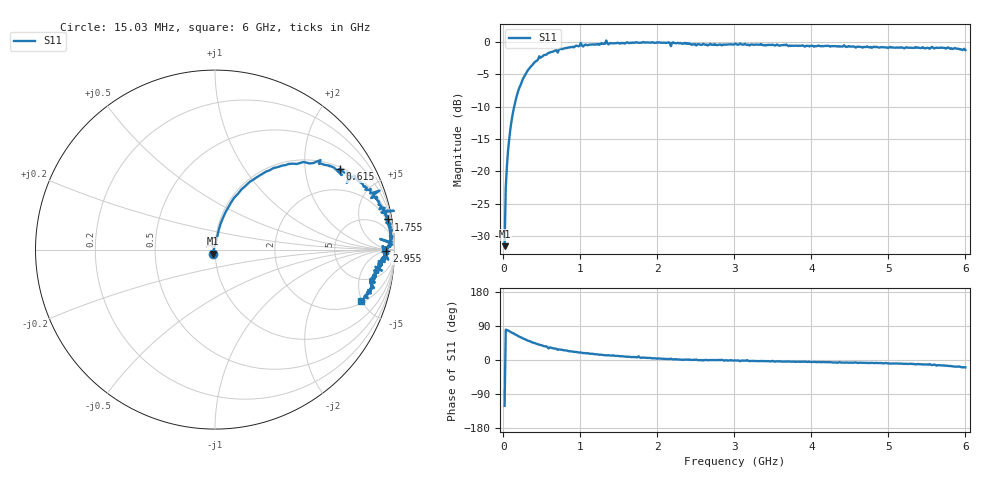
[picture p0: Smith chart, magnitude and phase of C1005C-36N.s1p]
!	Network	Analyzer	HP8753E.07.74:	Oct	30	2002	Serial	No.	JP38451487
!	Hewlett-Packard
!	7	Sep	2009	9:05:32
!	Frequency	S11
#	HZ	S	RI	R	50
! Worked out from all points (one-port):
!   400 points, 15.03 MHz to 6 GHz, reference 50 ohm
!   lowest |S11| = -31.5 dB at 15.03 MHz (marker M1), VSWR 1.05, Z = 48.6 - j2.22 ohm
!   |S11| at or under -10 dB: start of sweep to 139.9 MHz
!   S11 on the Smith chart (normalised r, x): 15.03 MHz: 0.97, -0.04; 615 MHz: 1.06, +3.06; 1.755 GHz: 1, +11; 2.955 GHz: 41, -7; 6 GHz: 2.19, -4.85
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1.502992e7  -0.0137 -0.0228
3.002985e7  0.0129 0.0734
6.00297e7  0.0305 0.142
1.050295e8  0.0736 0.234
1.650292e8  0.148 0.336
3.450283e8  0.409 0.477
4.650277e8  0.588 0.499
6.150269e8  0.698 0.45
7.650262e8  0.78 0.397
1.005025e9  0.917 0.329
1.035025e9  0.87 0.287
1.320023e9  0.939 0.217
1.335023e9  0.997 0.216
1.365023e9  0.928 0.206
1.515022e9  0.95 0.168
1.740021e9  0.975 0.121
1.755021e9  0.964 0.168
1.785021e9  0.977 0.0978
2.145019e9  0.986 0.0439
2.175019e9  0.92 0.0591
2.205019e9  0.987 0.0274
2.265019e9  0.978 0.0276
2.955015e9  0.954 -0.00763
3.015015e9  0.966 -0.0225
3.765011e9  0.925 -0.0649
4.515007e9  0.911 -0.108
5.265004e9  0.883 -0.16
6e9  0.811 -0.288
